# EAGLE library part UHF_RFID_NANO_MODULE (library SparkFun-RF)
UHF 860 and 920MHz RFID Module from ThingMagic
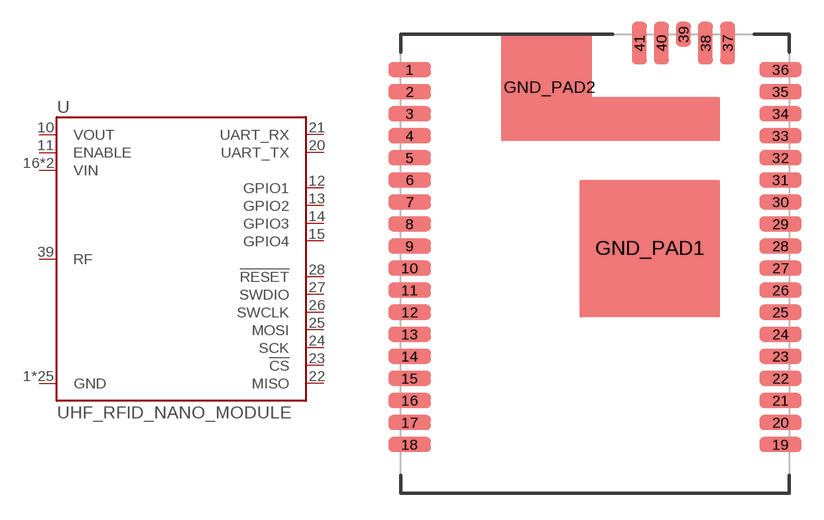
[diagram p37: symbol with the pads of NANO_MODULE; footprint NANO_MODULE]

Designator prefix U

## UHF_RFID_NANO_MODULE (PROD_ID: IC-13540; VALUE: Nano)  [NANO_MODULE]
1  GND
2  GND
3  GND
4  GND
5  GND
6  GND
7  GND
8  GND
9  GND
10  VOUT
11  ENABLE
12  GPIO1
13  GPIO2
14  GPIO3
15  GPIO4
16  VIN
17  VIN
18  GND
19  GND
20  UART_TX
21  UART_RX
22  MISO
23  !CS
24  SCK
25  MOSI
26  SWCLK
27  SWDIO
28  !RESET
29  GND
30  GND
31  GND
32  GND
33  GND
34  GND
35  GND
36  GND
37  GND
38  GND
39  RF
40  GND
41  GND
GND_PAD1  GND
GND_PAD2  GND

## Footprint NANO_MODULE (pad centres in mm)
smd 2.4 x 0.85: 1 -10.5,11; 2 -10.5,9.75; 3 -10.5,8.5; 4 -10.5,7.25; 5 -10.5,6; 6 -10.5,4.75; 7 -10.5,3.5; 8 -10.5,2.25; 9 -10.5,1; 10 -10.5,-0.25; 11 -10.5,-1.5; 12 -10.5,-2.75; 13 -10.5,-4; 14 -10.5,-5.25; 15 -10.5,-6.5; 16 -10.5,-7.75; 17 -10.5,-9; 18 -10.5,-10.25; 19 10.5,-10.25; 20 10.5,-9; 21 10.5,-7.75; 22 10.5,-6.5; 23 10.5,-5.25; 24 10.5,-4; 25 10.5,-2.75; 26 10.5,-1.5; 27 10.5,-0.25; 28 10.5,1; 29 10.5,2.25; 30 10.5,3.5; 31 10.5,4.75; 32 10.5,6; 33 10.5,7.25; 34 10.5,8.5; 35 10.5,9.75; 36 10.5,11
smd 0.85 x 2.4: 37 7.5,12.5; 38 6.25,12.5; 40 3.75,12.5; 41 2.5,12.5
smd 0.85 x 1.4: 39 5,13
smd 5 x 5: GND_PAD1 3.1,0.9
smd 4 x 4: GND_PAD2 -2.6,10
